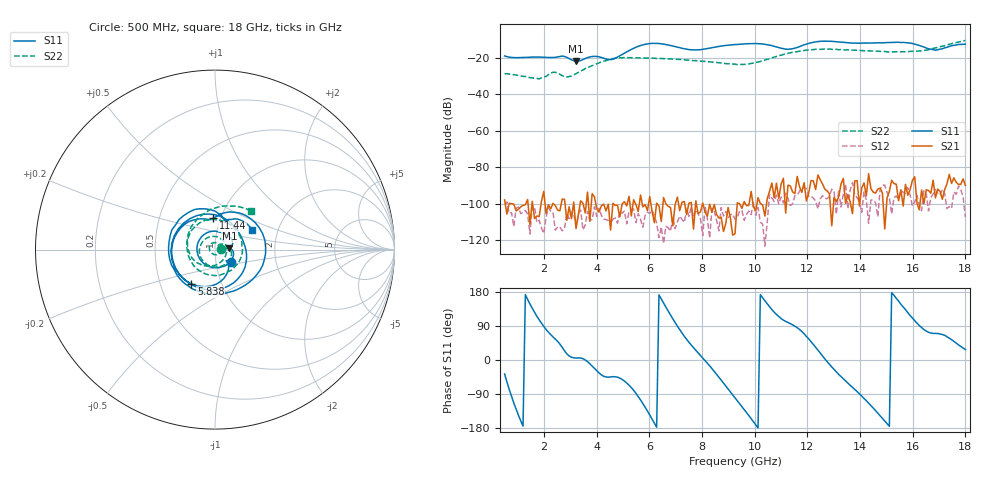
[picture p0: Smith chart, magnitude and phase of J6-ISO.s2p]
!Agilent Technologies,N5230A,MY45001360,A.07.50.67
!Agilent N5230A: A.07.50.67
!Date: Tuesday, April 16, 2024 16:01:04
!Correction: S11(Full 2 Port(1,2))
!S21(Full 2 Port(1,2))
!S12(Full 2 Port(1,2))
!S22(Full 2 Port(1,2))
!S2P File: Measurements: S11, S21, S12, S22:
# Hz S  dB  R 50
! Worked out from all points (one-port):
!   201 points, 500 MHz to 18 GHz, reference 50 ohm
!   lowest |S11| = -21.9 dB at 3.212 GHz (marker M1), VSWR 1.17, Z = 58.7 + j0.865 ohm
!   |S11| at or under -10 dB: start of sweep to end of sweep
!   S11 on the Smith chart (normalised r, x): 500 MHz: 1.18, -0.16; 5.838 GHz: 0.72, -0.29; 11.44 GHz: 0.92, +0.33; 18 GHz: 1.48, +0.34
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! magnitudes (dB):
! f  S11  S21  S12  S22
! 500 MHz  -19.1  -97.9  -100.7  -28.8
! 937.5 MHz  -20.0  -103.9  -102.4  -29.5
! 1.812 GHz  -19.7  -107.0  -108.9  -31.6
! 2.337 GHz  -19.9  -99.8  -104.5  -28.0
! 2.688 GHz  -19.1  -97.4  -114.8  -29.9
! 2.862 GHz  -19.8  -109.1  -105.1  -30.6
! 3.212 GHz  -21.9  -113.6  -112.3  -28.8
! 3.475 GHz  -21.0  -99.7  -114.2  -26.8
! 3.913 GHz  -19.3  -96.2  -101.7  -23.9
! 4.612 GHz  -20.9  -99.8  -108.3  -20.5
! 5.838 GHz  -12.7  -100.4  -106.4  -20.2
! 6.362 GHz  -12.3  -101.2  -118.5  -20.5
! 7.675 GHz  -15.8  -113.8  -107.0  -21.6
! 9.25 GHz  -12.8  -116.4  -108.5  -23.6
! 9.95 GHz  -12.3  -101.4  -99.4  -23.0
! 11.18 GHz  -15.4  -105.1  -94.2  -18.0
! 11.44 GHz  -15.1  -93.5  -100.0  -17.1
! 12.22 GHz  -11.6  -87.4  -96.9  -15.6
! 15.11 GHz  -11.7  -93.1  -96.7  -16.9
! 15.9 GHz  -12.0  -92.2  -95.1  -16.6
! 16.86 GHz  -15.9  -96.8  -92.3  -14.6
! 18 GHz  -12.6  -89.9  -107.4  -10.6
